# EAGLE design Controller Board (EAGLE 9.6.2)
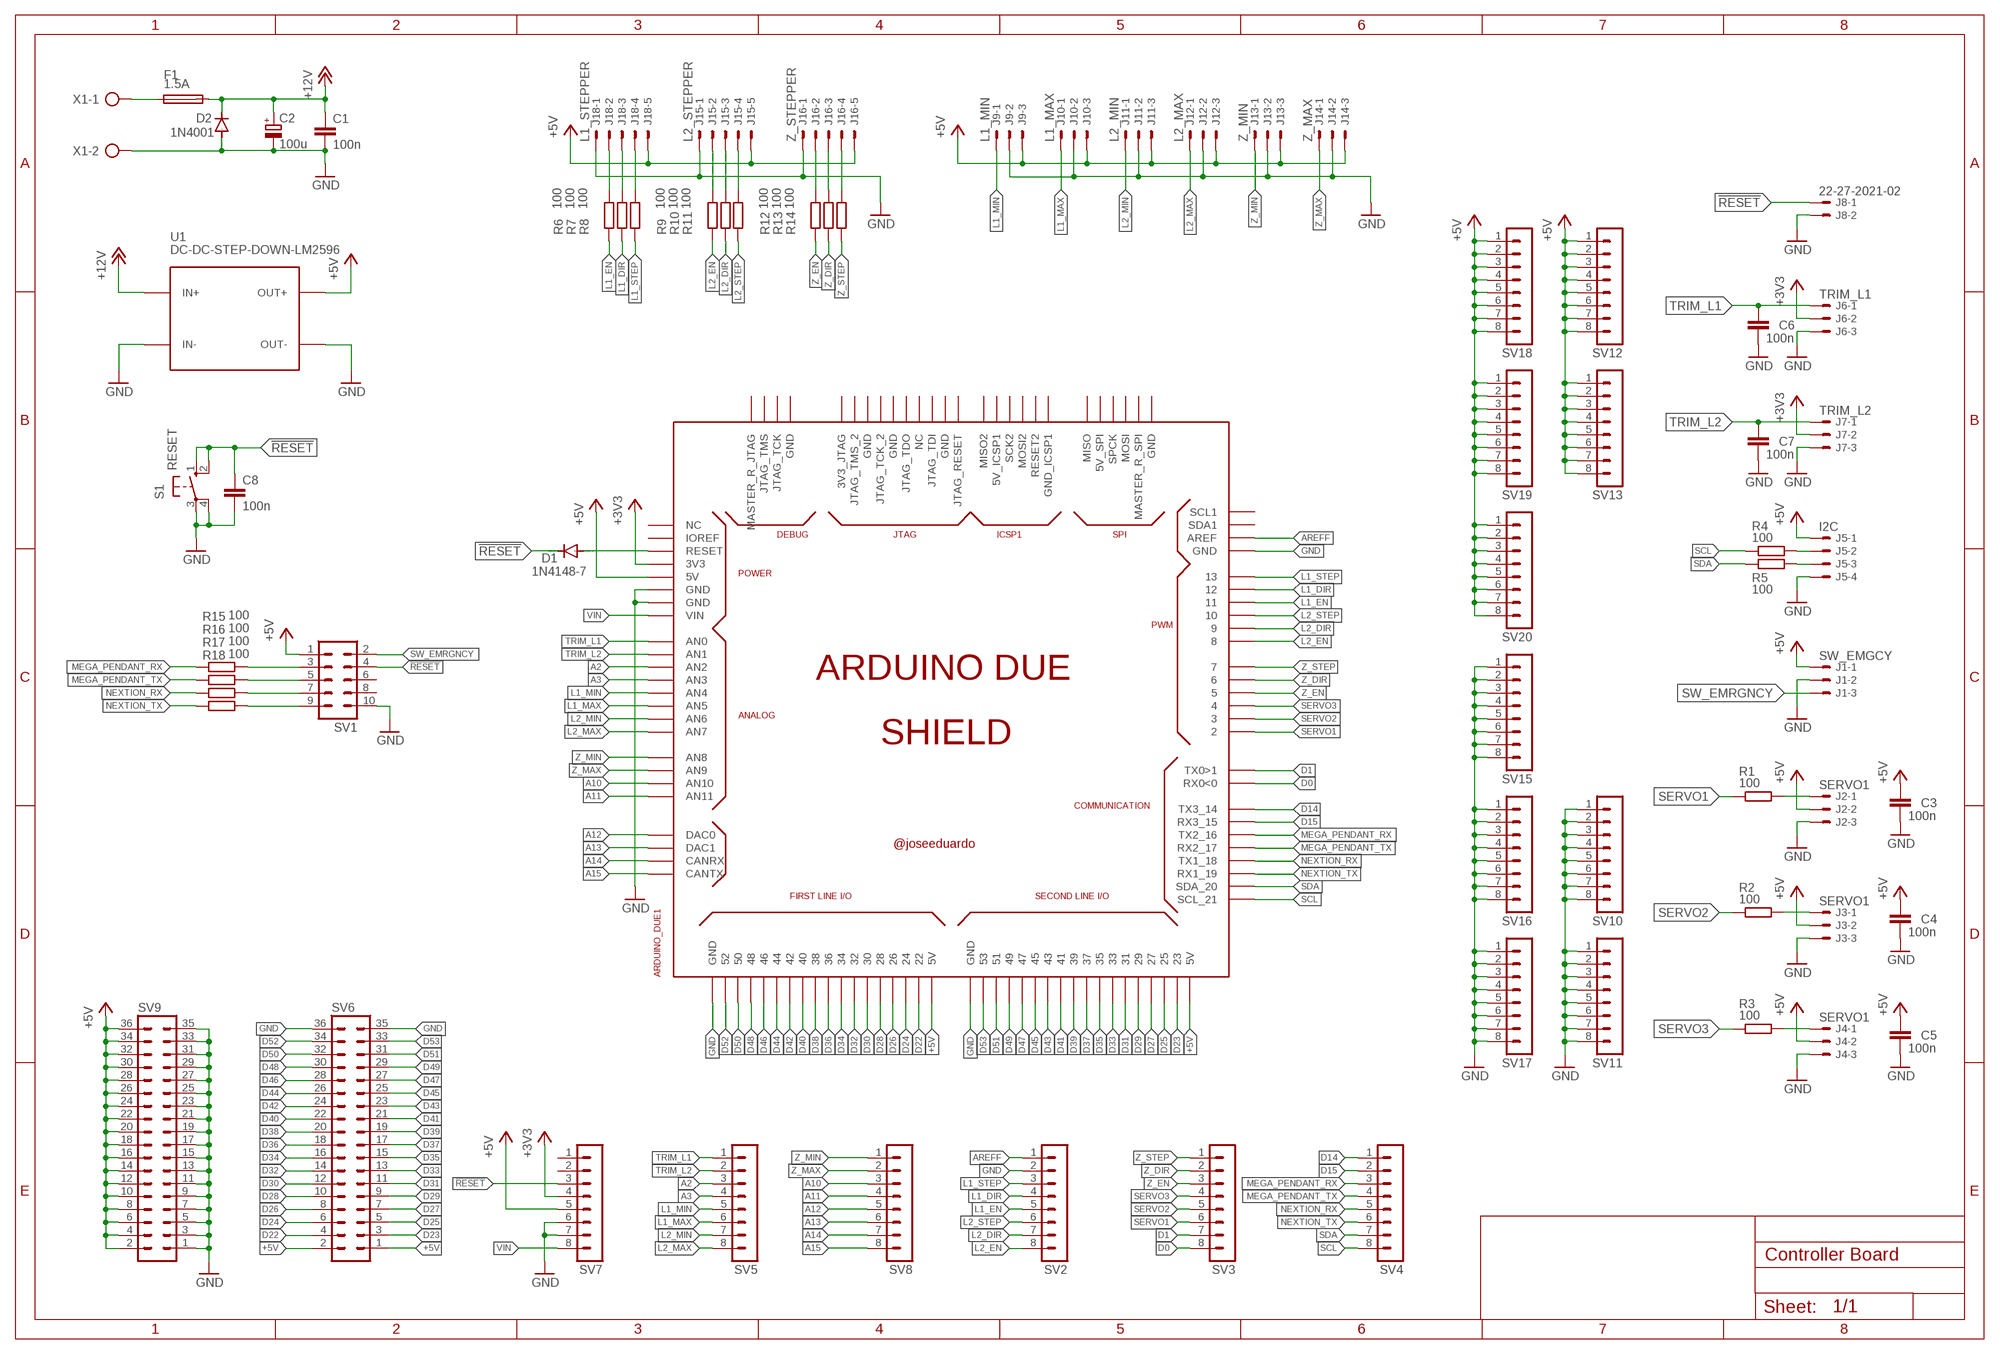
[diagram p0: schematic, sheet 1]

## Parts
ARDUINO_DUE1  ARDUINO_DUE_SHIELD_BTM  [ARDUINO_DUE_SHIELD_BOTTOM]
C1  100n  C-EU050-030X075  [C050-030X075]
C2  100u  CPOL-EUE3.5-8  [E3,5-8]
C3  100n  C-EU050-030X075  [C050-030X075]
C4  100n  C-EU050-030X075  [C050-030X075]
C5  100n  C-EU050-030X075  [C050-030X075]
C6  100n  C-EU050-030X075  [C050-030X075]
C7  100n  C-EU050-030X075  [C050-030X075]
C8  100n  C-EU050-030X075  [C050-030X075]
D1  1N4148-7  [DO35-7]
D2  1N4001  DIODE-DO41-7.6  [DO41-7.6]
F1  1.5A  SH22,5A  [SH22,5A]
J1  SW_EMGCY  22-27-2031-03  [6410-03]
J2  SERVO1  22-27-2031-03  [6410-03]
J3  SERVO1  22-27-2031-03  [6410-03]
J4  SERVO1  22-27-2031-03  [6410-03]
J5  I2C  22-27-2041-04  [6410-04]
J6  TRIM_L1  22-27-2031-03  [6410-03]
J7  TRIM_L2  22-27-2031-03  [6410-03]
J8  22-27-2021-02  [6410-02]
J9  L1_MIN  22-27-2031-03  [6410-03]
J10  L1_MAX  22-27-2031-03  [6410-03]
J11  L2_MIN  22-27-2031-03  [6410-03]
J12  L2_MAX  22-27-2031-03  [6410-03]
J13  Z_MIN  22-27-2031-03  [6410-03]
J14  Z_MAX  22-27-2031-03  [6410-03]
J15  L2_STEPPER  22-27-2051-05  [6410-05]
J16  Z_STEPPER  22-27-2051-05  [6410-05]
J18  L1_STEPPER  22-27-2051-05  [6410-05]
R1  100  R-EU_0207/7  [0207/7]
R2  100  R-EU_0207/7  [0207/7]
R3  100  R-EU_0207/7  [0207/7]
R4  100  R-EU_0207/7  [0207/7]
R5  100  R-EU_0207/7  [0207/7]
R6  100  R-EU_0207/7  [0207/7]
R7  100  R-EU_0207/7  [0207/7]
R8  100  R-EU_0207/7  [0207/7]
R9  100  R-EU_0207/7  [0207/7]
R10  100  R-EU_0207/7  [0207/7]
R11  100  R-EU_0207/7  [0207/7]
R12  100  R-EU_0207/7  [0207/7]
R13  100  R-EU_0207/7  [0207/7]
R14  100  R-EU_0207/7  [0207/7]
R15  100  R-EU_0207/7  [0207/7]
R16  100  R-EU_0207/7  [0207/7]
R17  100  R-EU_0207/7  [0207/7]
R18  100  R-EU_0207/7  [0207/7]
S1  RESET  10-XX  [B3F-10XX]
SV1  ML10  [ML10]
SV2  MA08-1  [MA08-1]
SV3  MA08-1  [MA08-1]
SV4  MA08-1  [MA08-1]
SV5  MA08-1  [MA08-1]
SV6  MA18-2  [MA18-2]
SV7  MA08-1  [MA08-1]
SV8  MA08-1  [MA08-1]
SV9  MA18-2  [MA18-2]
SV10  MA08-1  [MA08-1]
SV11  MA08-1  [MA08-1]
SV12  MA08-1  [MA08-1]
SV13  MA08-1  [MA08-1]
SV15  MA08-1  [MA08-1]
SV16  MA08-1  [MA08-1]
SV17  MA08-1  [MA08-1]
SV18  MA08-1  [MA08-1]
SV19  MA08-1  [MA08-1]
SV20  MA08-1  [MA08-1]
U1  DC-DC-STEP-DOWN-LM2596  [DC-DC-STEP-DOWN-LM2596]
X1  AK500/2  [AK500/2]

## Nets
!RESET: C8.1 D1.C J8.1 S1.1(S) S1.2(S1) SV1.4 SV7.3
+3V3: ARDUINO_DUE1.3V3 J6.2 J7.2 SV7.4
+5V: ARDUINO_DUE1.5V0(5V) ARDUINO_DUE1.5V0_1(5V) ARDUINO_DUE1.5V0_2(5V) C3.1 C4.1 C5.1 J1.1 J2.2 J3.2 J4.2 J5.1 J9.3 J10.3 J11.3 J12.3 J13.3 J14.3 J15.5 J16.5 J18.5 SV1.1 SV6.1 SV6.2 SV7.5 SV9.2 SV9.4 SV9.6 SV9.8 SV9.10 SV9.12 SV9.14 SV9.16 SV9.18 SV9.20 SV9.22 SV9.24 SV9.26 SV9.28 SV9.30 SV9.32 SV9.34 SV9.36 SV12.1 SV12.2 SV12.3 SV12.4 SV12.5 SV12.6 SV12.7 SV12.8 SV13.1 SV13.2 SV13.3 SV13.4 SV13.5 SV13.6 SV13.7 SV13.8 SV18.1 SV18.2 SV18.3 SV18.4 SV18.5 SV18.6 SV18.7 SV18.8 SV19.1 SV19.2 SV19.3 SV19.4 SV19.5 SV19.6 SV19.7 SV19.8 SV20.1 SV20.2 SV20.3 SV20.4 SV20.5 SV20.6 SV20.7 SV20.8 U1.OUT+
+12V: C1.1 C2.+ D2.C F1.2 U1.IN+
A2: ARDUINO_DUE1.A2(AN2) SV5.3
A3: ARDUINO_DUE1.A3(AN3) SV5.4
A10: ARDUINO_DUE1.A10(AN10) SV8.3
A11: ARDUINO_DUE1.A11(AN11) SV8.4
A12: ARDUINO_DUE1.DAC0 SV8.5
A13: ARDUINO_DUE1.DAC1 SV8.6
A14: ARDUINO_DUE1.CANRX SV8.7
A15: ARDUINO_DUE1.CANTX SV8.8
AREFF: ARDUINO_DUE1.AREF SV2.1
D0: ARDUINO_DUE1.0(RX0<0) SV3.8
D1: ARDUINO_DUE1.1(TX0>1) SV3.7
D14: ARDUINO_DUE1.14(TX3_14) SV4.1
D15: ARDUINO_DUE1.15(RX3_15) SV4.2
D22: ARDUINO_DUE1.22 SV6.4
D23: ARDUINO_DUE1.23 SV6.3
D24: ARDUINO_DUE1.24 SV6.6
D25: ARDUINO_DUE1.25 SV6.5
D26: ARDUINO_DUE1.26 SV6.8
D27: ARDUINO_DUE1.27 SV6.7
D28: ARDUINO_DUE1.28 SV6.10
D29: ARDUINO_DUE1.29 SV6.9
D30: ARDUINO_DUE1.30 SV6.12
D31: ARDUINO_DUE1.31 SV6.11
D32: ARDUINO_DUE1.32 SV6.14
D33: ARDUINO_DUE1.33 SV6.13
D34: ARDUINO_DUE1.34 SV6.16
D35: ARDUINO_DUE1.35 SV6.15
D36: ARDUINO_DUE1.36 SV6.18
D37: ARDUINO_DUE1.37 SV6.17
D38: ARDUINO_DUE1.38 SV6.20
D39: ARDUINO_DUE1.39 SV6.19
D40: ARDUINO_DUE1.40 SV6.22
D41: ARDUINO_DUE1.41 SV6.21
D42: ARDUINO_DUE1.42 SV6.24
D43: ARDUINO_DUE1.43 SV6.23
D44: ARDUINO_DUE1.44 SV6.26
D45: ARDUINO_DUE1.45 SV6.25
D46: ARDUINO_DUE1.46 SV6.28
D47: ARDUINO_DUE1.47 SV6.27
D48: ARDUINO_DUE1.48 SV6.30
D49: ARDUINO_DUE1.49 SV6.29
D50: ARDUINO_DUE1.50 SV6.32
D51: ARDUINO_DUE1.51 SV6.31
D52: ARDUINO_DUE1.52 SV6.34
D53: ARDUINO_DUE1.53 SV6.33
GND: ARDUINO_DUE1.GND ARDUINO_DUE1.GND_1(GND) ARDUINO_DUE1.GND_2(GND) ARDUINO_DUE1.GND_3(GND) ARDUINO_DUE1.GND_4(GND) C1.2 C2.- C3.2 C4.2 C5.2 C6.2 C7.2 C8.2 D2.A J1.2 J2.3 J3.3 J4.3 J5.4 J6.3 J7.3 J8.2 J9.2 J10.2 J11.2 J12.2 J13.2 J14.2 J15.1 J16.1 J18.1 S1.3(P) S1.4(P1) SV1.10 SV2.2 SV6.35 SV6.36 SV7.6 SV7.7 SV9.1 SV9.3 SV9.5 SV9.7 SV9.9 SV9.11 SV9.13 SV9.15 SV9.17 SV9.19 SV9.21 SV9.23 SV9.25 SV9.27 SV9.29 SV9.31 SV9.33 SV9.35 SV10.1 SV10.2 SV10.3 SV10.4 SV10.5 SV10.6 SV10.7 SV10.8 SV11.1 SV11.2 SV11.3 SV11.4 SV11.5 SV11.6 SV11.7 SV11.8 SV15.1 SV15.2 SV15.3 SV15.4 SV15.5 SV15.6 SV15.7 SV15.8 SV16.1 SV16.2 SV16.3 SV16.4 SV16.5 SV16.6 SV16.7 SV16.8 SV17.1 SV17.2 SV17.3 SV17.4 SV17.5 SV17.6 SV17.7 SV17.8 U1.IN- U1.OUT- X1.2
L1_DIR: ARDUINO_DUE1.12 R7.1 SV2.4
L1_EN: ARDUINO_DUE1.11 R6.1 SV2.5
L1_MAX: ARDUINO_DUE1.A5(AN5) J10.1 SV5.6
L1_MIN: ARDUINO_DUE1.A4(AN4) J9.1 SV5.5
L1_STEP: ARDUINO_DUE1.13 R8.1 SV2.3
L2_DIR: ARDUINO_DUE1.9 R10.1 SV2.7
L2_EN: ARDUINO_DUE1.8 R9.1 SV2.8
L2_MAX: ARDUINO_DUE1.A7(AN7) J12.1 SV5.8
L2_MIN: ARDUINO_DUE1.A6(AN6) J11.1 SV5.7
L2_STEP: ARDUINO_DUE1.10 R11.1 SV2.6
MEGA_PENDANT_RX: ARDUINO_DUE1.16(TX2_16) R15.1 SV4.3
MEGA_PENDANT_TX: ARDUINO_DUE1.17(RX2_17) R16.1 SV4.4
N$1: ARDUINO_DUE1.RESET D1.A
N$2: F1.1 X1.1
N$3: J2.1 R1.2
N$4: J3.1 R2.2
N$5: J4.1 R3.2
N$6: J5.2 R4.2
N$7: J5.3 R5.2
N$8: J18.2 R6.2
N$9: J18.3 R7.2
N$10: J18.4 R8.2
N$11: J15.2 R9.2
N$12: J15.3 R10.2
N$13: J15.4 R11.2
N$14: J16.4 R14.2
N$15: J16.3 R13.2
N$16: J16.2 R12.2
N$17: R15.2 SV1.3
N$18: R16.2 SV1.5
N$19: R17.2 SV1.7
N$20: R18.2 SV1.9
NEXTION_RX: ARDUINO_DUE1.18(TX1_18) R17.1 SV4.5
NEXTION_TX: ARDUINO_DUE1.19(RX1_19) R18.1 SV4.6
SCL: ARDUINO_DUE1.21(SCL_21) R4.1 SV4.8
SDA: ARDUINO_DUE1.20(SDA_20) R5.1 SV4.7
SERVO1: ARDUINO_DUE1.2 R1.1 SV3.6
SERVO2: ARDUINO_DUE1.3 R2.1 SV3.5
SERVO3: ARDUINO_DUE1.4 R3.1 SV3.4
SW_EMRGNCY: J1.3 SV1.2
TRIM_L1: ARDUINO_DUE1.A0(AN0) C6.1 J6.1 SV5.1
TRIM_L2: ARDUINO_DUE1.A1(AN1) C7.1 J7.1 SV5.2
VIN: ARDUINO_DUE1.VIN SV7.8
Z_DIR: ARDUINO_DUE1.6 R13.1 SV3.2
Z_EN: ARDUINO_DUE1.5 R12.1 SV3.3
Z_MAX: ARDUINO_DUE1.A9(AN9) J14.1 SV8.2
Z_MIN: ARDUINO_DUE1.A8(AN8) J13.1 SV8.1
Z_STEP: ARDUINO_DUE1.7 R14.1 SV3.1
Unconnected: ARDUINO_DUE1.3V3_JTAG ARDUINO_DUE1.5V_2(5V_SPI) ARDUINO_DUE1.5V_ICSP1 ARDUINO_DUE1.GND_5(GND) ARDUINO_DUE1.GND_7(GND) ARDUINO_DUE1.GND_8(GND) ARDUINO_DUE1.GND_9(GND) ARDUINO_DUE1.GND_10(GND) ARDUINO_DUE1.GND_ICSP1 ARDUINO_DUE1.IOREF ARDUINO_DUE1.JTAG_RESET ARDUINO_DUE1.JTAG_TCK ARDUINO_DUE1.JTAG_TCK_2 ARDUINO_DUE1.JTAG_TDI ARDUINO_DUE1.JTAG_TDO ARDUINO_DUE1.JTAG_TMS ARDUINO_DUE1.JTAG_TMS_2 ARDUINO_DUE1.MASTER_RESET_JTAG(MASTER_R_JTAG) ARDUINO_DUE1.MASTER_RESET_SPI(MASTER_R_SPI) ARDUINO_DUE1.MISO ARDUINO_DUE1.MISO2 ARDUINO_DUE1.MOSI ARDUINO_DUE1.MOSI2 ARDUINO_DUE1.NC_2(NC) ARDUINO_DUE1.NC_5(NC) ARDUINO_DUE1.RESET2 ARDUINO_DUE1.SCK2 ARDUINO_DUE1.SCL1 ARDUINO_DUE1.SDA1 ARDUINO_DUE1.SPCK SV1.6 SV1.8 SV7.1 SV7.2

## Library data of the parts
ARDUINO_DUE1 = arduino_due_shield:ARDUINO_DUE_SHIELD
C1 C3-C8 = rcl:C-EU: CAPACITOR, European symbol; SPICEPREFIX: C
C2 = rcl:CPOL-EU: POLARIZED CAPACITOR, European symbol; SPICEPREFIX: C
D1 = diode:1N4148: DIODE
D2 = diode:DIODE-: DIODE
F1 = Khoirul_Component:SH22,5A: FUSE HOLDER
J1-J4 J6 J7 J9-J14 = con-molex:22-?-03: CONNECTOR wire to board 2.54 mm (.1 inch) pitch header; MF: MOLEX; OC_FARNELL: unknown; OC_NEWARK: unknown
J5 = con-molex:22-?-04: CONNECTOR wire to board 2.54 mm (.1 inch) pitch header; MF: MOLEX; OC_FARNELL: unknown; OC_NEWARK: unknown
J8 = con-molex:22-?-02: CONNECTOR; MF: MOLEX; OC_FARNELL: unknown; OC_NEWARK: unknown
J15 J16 J18 = con-molex:22-?-05: CONNECTOR wire to board 2.54 mm (.1 inch) pitch header; MF: MOLEX; OC_FARNELL: unknown; OC_NEWARK: unknown
R1-R18 = rcl:R-EU_: RESISTOR, European symbol; SPICEPREFIX: R
S1 = switch-omron:10-XX: OMRON SWITCH; MPN: B3F-1000; OC_FARNELL: 176432; OC_NEWARK: 36M3542
SV1 = con-ml:ML10: HARTING; OC_FARNELL: unknown; OC_NEWARK: unknown
SV2-SV5 SV7 SV8 SV10-SV13 SV15-SV20 = con-lstb:MA08-1: PIN HEADER; OC_FARNELL: unknown; OC_NEWARK: unknown
SV6 SV9 = con-lstb:MA18-2: PIN HEADER; OC_FARNELL: unknown; OC_NEWARK: unknown
U1 = diy-modules:DC-DC-STEP-DOWN-LM2596: DC/DC Step-Down Regulator based on LM2596-ADJ chip LM2596 datasheet available here: http://www.ti.com/lit/ds/symlink/lm2596.pdf Click here to find device on ebay.com
X1 = con-ptr500:AK500/2: CONNECTOR; OC_FARNELL: unknown; OC_NEWARK: unknown

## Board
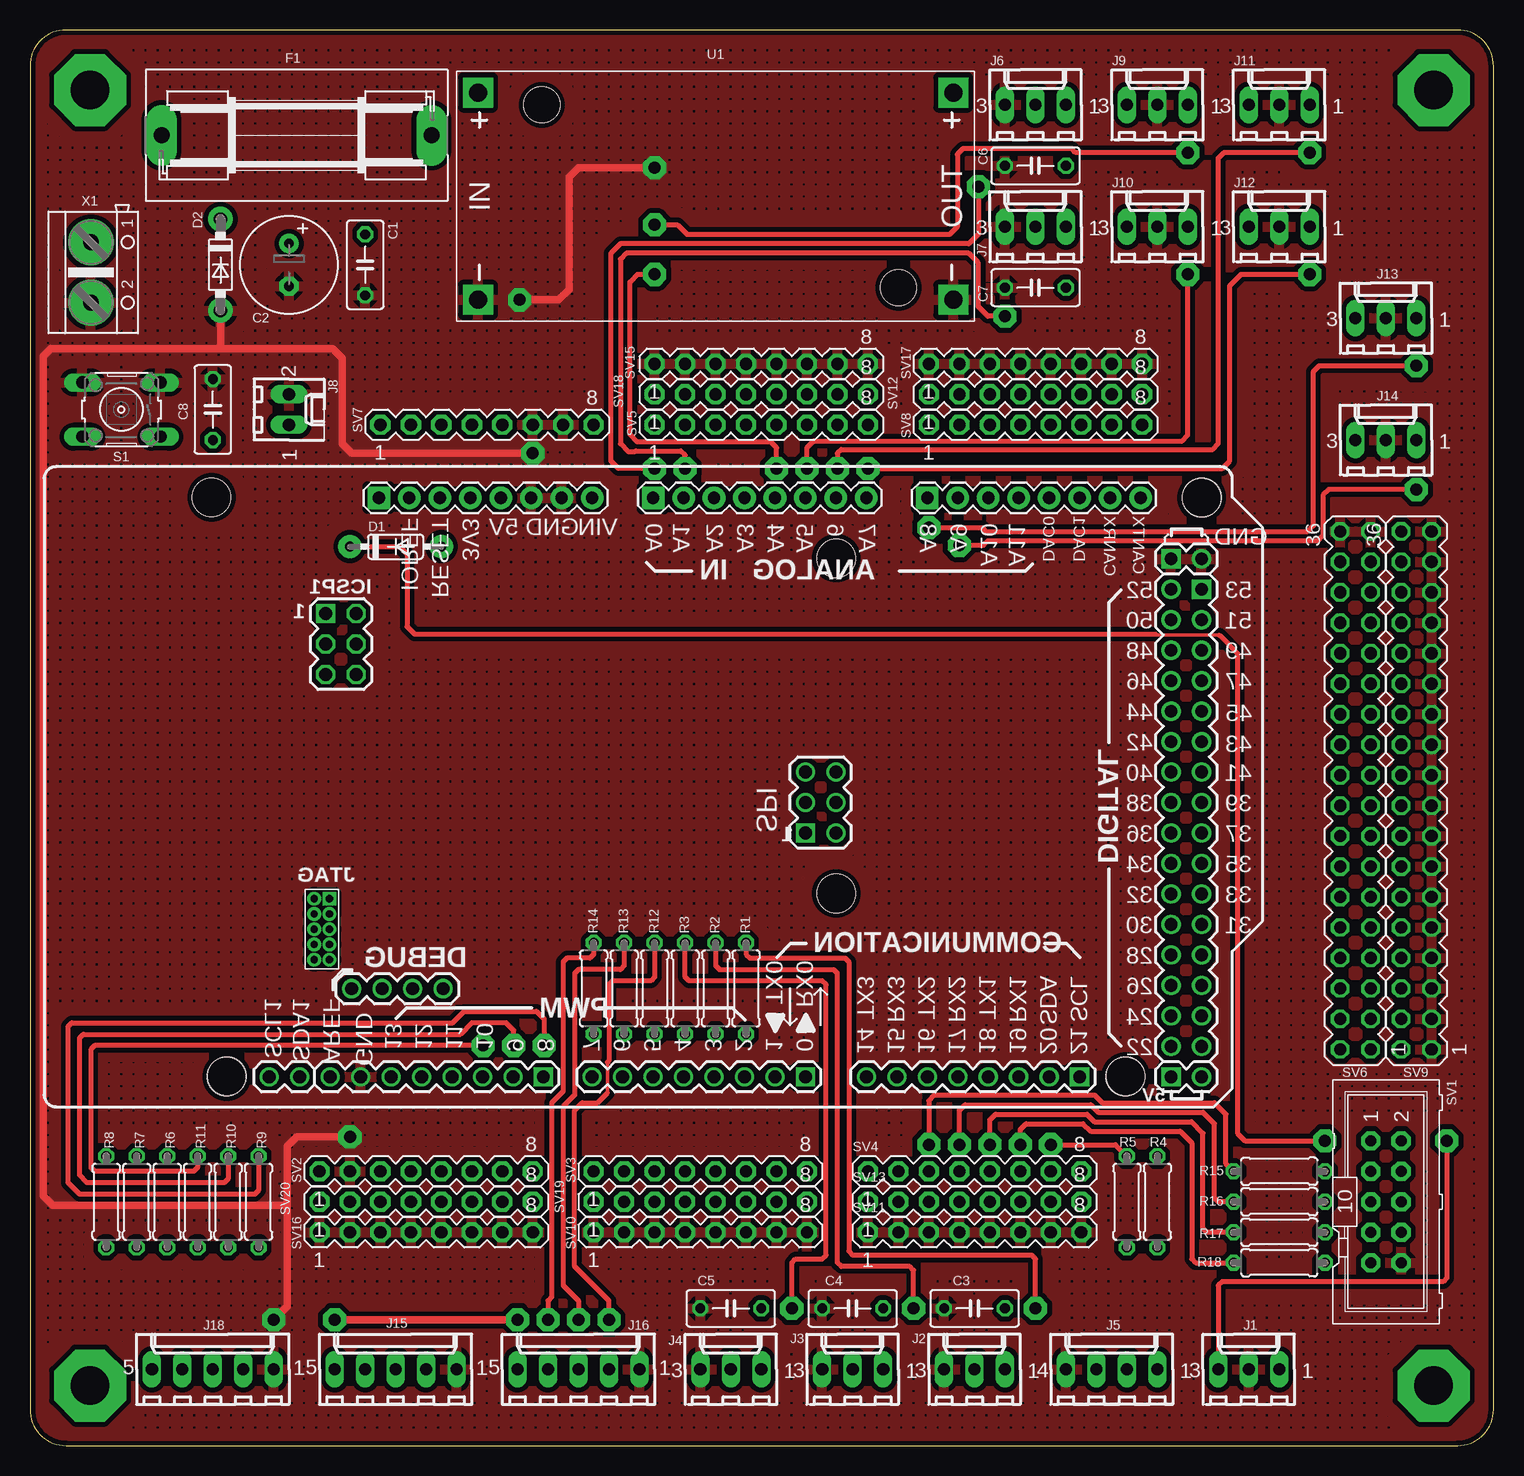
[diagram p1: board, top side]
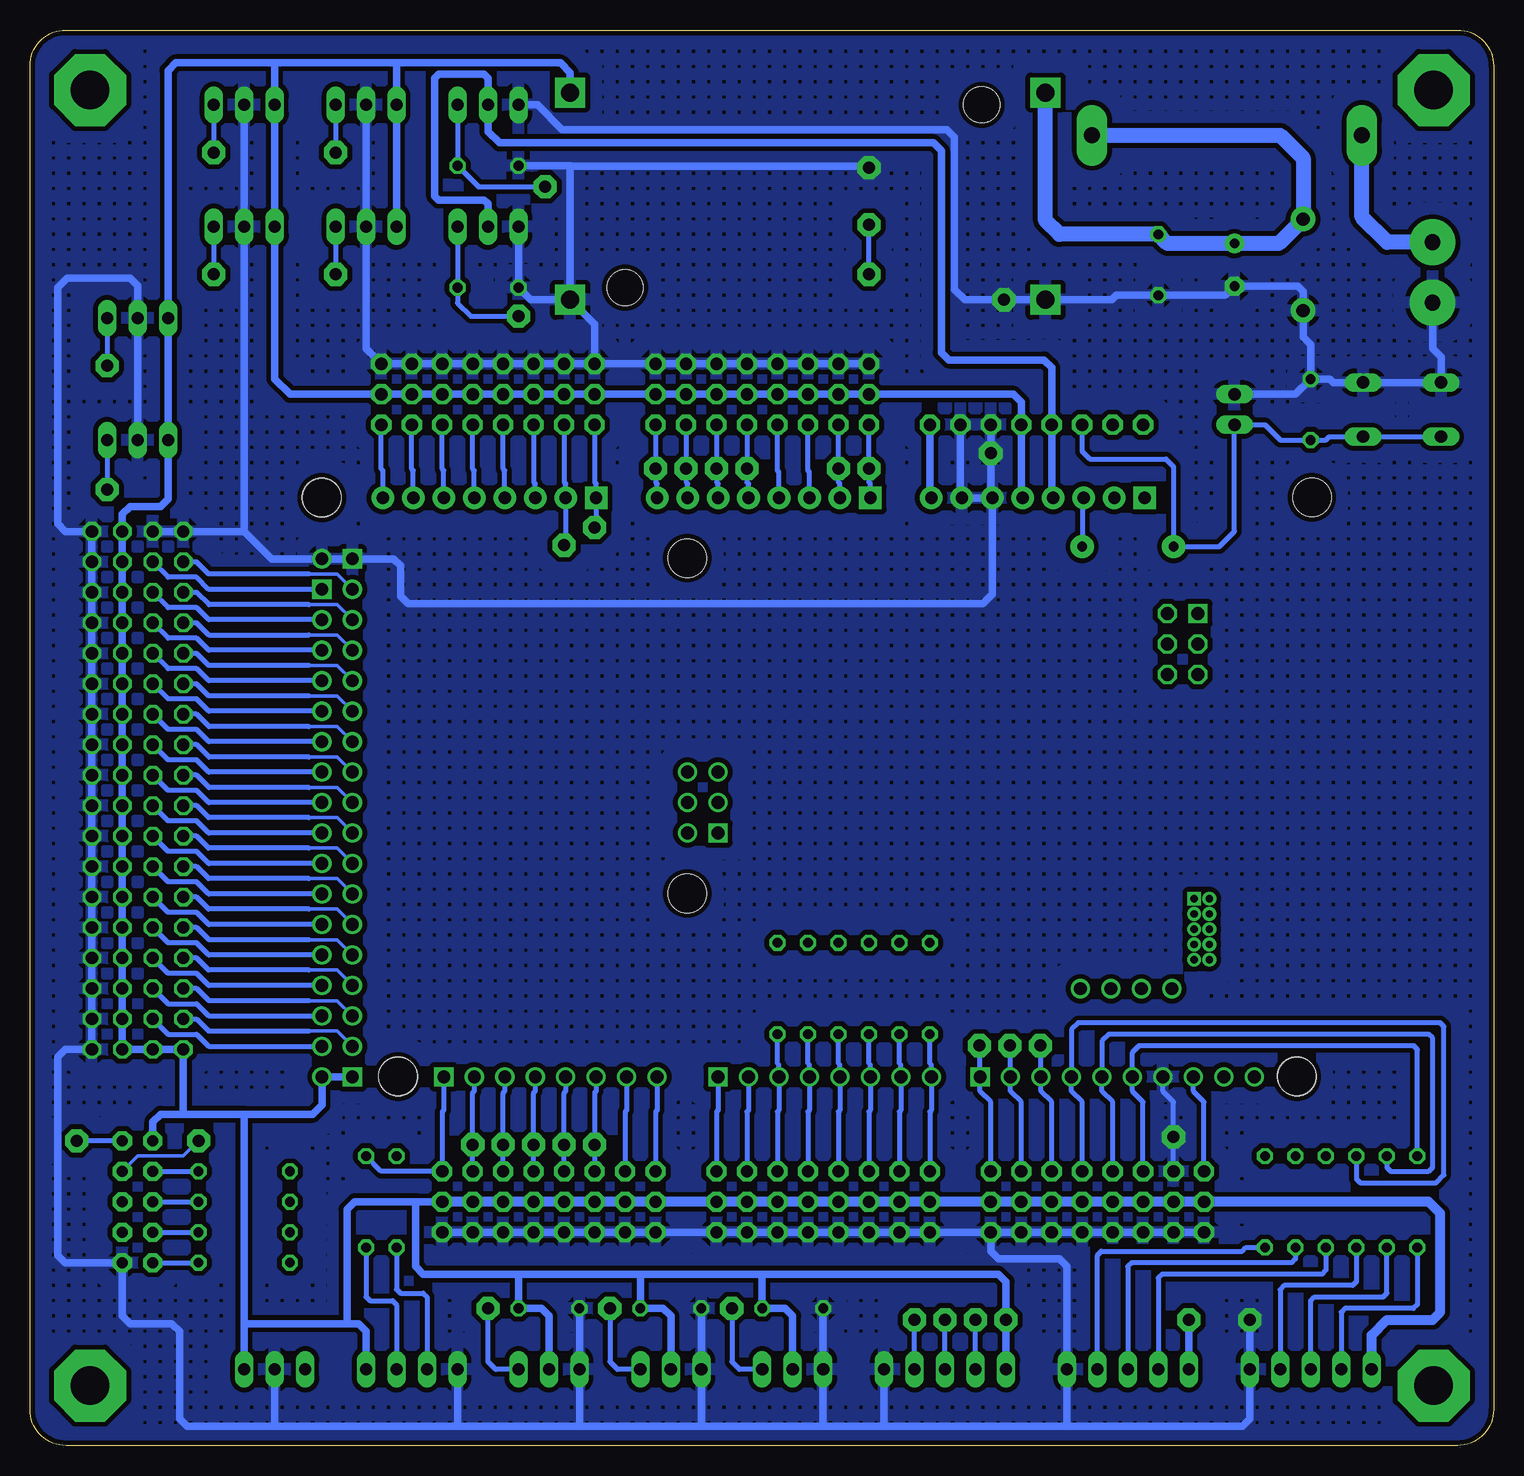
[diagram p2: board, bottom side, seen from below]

Size 122 x 118 mm. Coordinates in mm from the lower left corner, seen from the top.
Outline: 122,3 122,115 arc90 119,118 3,118 arc90 0,115 0,3 arc90 3,0 119,0 arc90 122,3
Copper layers (1*16): Top 0.035mm / dielectric 1.5mm / Bottom 0.035mm
Design rules "default": minimum track width 12mil, minimum drill 0.8mm, track to track 12mil, track to pad 12mil, pad to pad 12mil, via to via 12mil, smd to smd 12mil, copper to edge 12mil, drill to drill 6mil, minimum pad ring 10mil, minimum via ring 8mil, stop-mask expansion 12mil, vias tented up to drill 0mil, thermal gap 16mil

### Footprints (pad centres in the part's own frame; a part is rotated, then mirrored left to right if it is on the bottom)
ARDUINO_DUE_SHIELD_BOTTOM = drill 1.067 square: 0 63.373,51.816; 5V0_1 93.853,51.816; 8 41.529,51.816; 21 86.233,51.816; 53 96.393,11.176; GND_2 93.853,8.636; MISO 63.373,31.496; MISO2 23.384,13.196 | drill 1.067: 1 60.833,51.816; 2 58.293,51.816; 3 55.753,51.816; 4 53.213,51.816; 5 50.673,51.816; 5V0_2 96.393,51.816; 5V_2 65.913,31.496; 6 48.133,51.816; 7 45.593,51.816; 9 38.989,51.816; 10 36.449,51.816; 11 33.909,51.816; 12 31.369,51.816; 13 28.829,51.816; 14 68.453,51.816; 15 70.993,51.816; 16 73.533,51.816; 17 76.073,51.816; 18 78.613,51.816; 19 81.153,51.816; 20 83.693,51.816; 22 93.853,49.276; 23 96.393,49.276; 24 93.853,46.736; 25 96.393,46.736; 26 93.853,44.196; 27 96.393,44.196; 28 93.853,41.656; 29 96.393,41.656; 30 93.853,39.116; 31 96.393,39.116; 32 93.853,36.576; 33 96.393,36.576; 34 93.853,34.036; 35 96.393,34.036; 36 93.853,31.496; 37 96.393,31.496; 38 93.853,28.956; 39 96.393,28.956; 40 93.853,26.416; 41 96.393,26.416; 42 93.853,23.876; 43 96.393,23.876; 44 93.853,21.336; 45 96.393,21.336; 46 93.853,18.796; 47 96.393,18.796; 48 93.853,16.256; 49 96.393,16.256; 50 93.853,13.716; 51 96.393,13.716; 52 93.853,11.176; AREF 23.749,51.816; GND_3 96.393,8.636; GND_4 26.289,51.816; GND_5 65.913,26.416; GND_7 33.161,44.473; JTAG_TCK 30.621,44.473; JTAG_TMS 28.081,44.473; MASTER_RESET_JTAG 25.541,44.473; MASTER_RESET_SPI 63.373,26.416; MOSI 65.913,28.956; SCL1 18.669,51.816; SDA1 21.209,51.816; SPCK 63.373,28.956 | drill 1.016 pad 1.88: 3V3 35.433,3.556; 5V0 37.973,3.556; A1 53.213,3.556; A2 55.753,3.556; A3 58.293,3.556; A4 60.833,3.556; A5 63.373,3.556; A6 65.913,3.556; A7 68.453,3.556; A9 76.073,3.556; A10 78.613,3.556; A11 81.153,3.556; CANRX 88.773,3.556; CANTX 91.313,3.556; DAC0 83.693,3.556; DAC1 86.233,3.556; GND 40.513,3.556; GND_1 43.053,3.556; IOREF 30.346,3.543; RESET 32.893,3.555; VIN 45.593,3.556 | drill 0.6 pad 1.016 square: 3V3_JTAG 23.689,36.964 | drill 1.067 octagon: 5V_ICSP1 25.924,13.196; GND_ICSP1 25.924,18.276; MOSI2 25.924,15.736; RESET2 23.384,18.276; SCK2 23.384,15.736 | drill 1.016 pad 1.88 square: A0 50.673,3.556; A8 73.533,3.556; NC_2 27.806,3.543 | drill 0.6 pad 1.143: GND_8 23.689,38.234; GND_9 23.689,40.774; GND_10 23.689,42.044; JTAG_RESET 22.419,42.044; JTAG_TCK_2 22.419,38.234; JTAG_TDI 22.419,40.774; JTAG_TDO 22.419,39.504; JTAG_TMS_2 22.419,36.964; NC_5 23.689,39.504 | hole 3.2: 15.113,51.816; 90.043,51.816; 96.393,3.556; 96.418,3.505; 15.138,51.765; 90.068,51.765; 13.868,3.505; 65.938,36.525; 65.938,8.585
C050-030X075 = drill 0.813 octagon: 1 -2.54,0; 2 2.54,0
E3,5-8 = drill 0.813 pad 1.6: + -1.778,0 | drill 0.813 pad 1.6 octagon: - 1.778,0
DO35-7 = drill 0.813 pad 1.93: A 3.81,0; C -3.81,0
DO41-7.6 = drill 1.1 pad 2.032: A 3.81,0; C -3.81,0
SH22,5A = drill 1.321 pad 2.54 long: 1 -11.252,0; 2 11.252,0
6410-03 = drill 1.016 long: 1 2.54,0; 2 0,0; 3 -2.54,0
6410-04 = drill 1.016 long: 1 3.81,0; 2 1.27,0; 3 -1.27,0; 4 -3.81,0
6410-02 = drill 1.016 long: 1 1.27,0; 2 -1.27,0
6410-05 = drill 1.016 long: 1 5.08,0; 2 2.54,0; 3 0,0; 4 -2.54,0; 5 -5.08,0
0207/7 = drill 0.813 octagon: 1 -3.81,0; 2 3.81,0
B3F-10XX = drill 1.016 long: 1 -3.251,2.261; 2 3.251,2.261; 3 -3.251,-2.261; 4 3.251,-2.261
ML10 = drill 0.914 pad 1.6 octagon: 1 -5.08,-1.27; 2 -5.08,1.27; 3 -2.54,-1.27; 4 -2.54,1.27; 5 0,-1.27; 6 0,1.27; 7 2.54,-1.27; 8 2.54,1.27; 9 5.08,-1.27; 10 5.08,1.27
MA08-1 = drill 1.016 pad 1.676 octagon: 1 -8.89,0; 2 -6.35,0; 3 -3.81,0; 4 -1.27,0; 5 1.27,0; 6 3.81,0; 7 6.35,0; 8 8.89,0
MA18-2 = drill 1.016 octagon: 1 -21.59,-1.27; 2 -21.59,1.27; 3 -19.05,-1.27; 4 -19.05,1.27; 5 -16.51,-1.27; 6 -16.51,1.27; 7 -13.97,-1.27; 8 -13.97,1.27; 9 -11.43,-1.27; 10 -11.43,1.27; 11 -8.89,-1.27; 12 -8.89,1.27; 13 -6.35,-1.27; 14 -6.35,1.27; 15 -3.81,-1.27; 16 -3.81,1.27; 17 -1.27,-1.27; 18 -1.27,1.27; 19 1.27,-1.27; 20 1.27,1.27; 21 3.81,-1.27; 22 3.81,1.27; 23 6.35,-1.27; 24 6.35,1.27; 25 8.89,-1.27; 26 8.89,1.27; 27 11.43,-1.27; 28 11.43,1.27; 29 13.97,-1.27; 30 13.97,1.27; 31 16.51,-1.27; 32 16.51,1.27; 33 19.05,-1.27; 34 19.05,1.27; 35 21.59,-1.27; 36 21.59,1.27
DC-DC-STEP-DOWN-LM2596 = drill 1.5 pad 2.5 square: IN+ -19.812,8.636; IN- -19.812,-8.636; OUT+ 19.812,8.636; OUT- 19.812,-8.636 | hole 3: -14.478,7.62; 15.24,-7.62
AK500/2 = drill 1.321 pad 3.81: 1 -2.515,0; 2 2.515,0

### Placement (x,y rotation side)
ARDUINO_DUE1  1.27,82.55 180 bottom
C1  27.94,98.42 270 top
C2  21.59,98.42 270 top
C3  78.74,11.43 180 top
C4  68.58,11.43 180 top
C5  58.42,11.43 180 top
C6  83.82,106.68 180 top
C7  83.82,96.52 180 top
C8  15.24,86.36 90 top
D1  30.48,74.93 0 top
D2  15.88,98.42 270 top
F1  22.23,109.22 0 top
J1  101.6,6.35 0 top
J2  78.74,6.35 0 top
J3  68.58,6.35 0 top
J4  58.42,6.35 0 top
J5  90.17,6.35 0 top
J6  83.82,111.76 0 top
J7  83.82,101.6 0 top
J8  21.59,86.36 270 top
J9  93.98,111.76 0 top
J10  93.98,101.6 0 top
J11  104.14,111.76 0 top
J12  104.14,101.6 0 top
J13  113.03,93.98 0 top
J14  113.03,83.82 0 top
J15  30.48,6.35 0 top
J16  45.72,6.35 0 top
J18  15.24,6.35 0 top
R1  59.69,38.1 90 top
R2  57.15,38.1 90 top
R3  54.61,38.1 90 top
R4  93.98,20.32 270 top
R5  91.44,20.32 270 top
R6  11.43,20.32 270 top
R7  8.89,20.32 270 top
R8  6.35,20.32 270 top
R9  19.05,20.32 270 top
R10  16.51,20.32 270 top
R11  13.97,20.32 270 top
R12  52.07,38.1 90 top
R13  49.53,38.1 90 top
R14  46.99,38.1 90 top
R15  104.14,22.86 0 top
R16  104.14,20.32 0 top
R17  104.14,17.78 0 top
R18  104.14,15.24 0 top
S1  7.62,86.36 180 top
SV1  113.03,20.32 270 top
SV2  33.02,22.86 0 top
SV3  55.88,22.86 0 top
SV4  78.74,22.86 0 top
SV5  60.96,85.09 0 top
SV6  110.49,54.61 90 top
SV7  38.1,85.09 0 top
SV8  83.82,85.09 0 top
SV9  115.57,54.61 90 top
SV10  55.88,17.78 0 top
SV11  78.74,17.78 0 top
SV12  83.82,87.63 0 top
SV13  78.74,20.32 0 top
SV15  60.96,90.17 0 top
SV16  33.02,17.78 0 top
SV17  83.82,90.17 0 top
SV18  60.96,87.63 0 top
SV19  55.88,20.32 0 top
SV20  33.02,20.32 0 top
U1  57.15,104.14 0 top
X1  5.08,97.79 270 top

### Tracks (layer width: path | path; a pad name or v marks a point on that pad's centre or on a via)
!RESET  (via drill 1 pad 1.93)
  Top 0.305: 93.82,67.63 93.9,67.55 99.14,67.55
  Top 0.406: 93.82,67.63 32.07,67.63 31.43,68.26 31.43,74.3 30.8,74.93 D1.C | 99.14,67.55 100.65,66.04 100.65,26.04 101.28,25.4 v107.95,25.4
  Bottom 0.305: SV1.4 113.03,24.13 109.22,24.13 v107.95,25.4
  Bottom 0.406: S1.2 S1.1 13.69,84.1 13.97,83.82 C8.1 17.78,83.82 19.05,85.09 J8.1 21.59,76.2 22.86,74.93 D1.C 26.67,81.6 27.3,82.23 33.66,82.23 34.29,82.87 SV7.3
+3V3
  Bottom 0.61: ARDUINO_DUE1.3V3 36.83,79.12 SV7.4 36.83,89.85 37.47,90.49 45.4,90.49 46.04,91.12 46.04,107.95 46.67,108.58 82.87,108.58 83.82,109.54 J6.2 83.82,113.98 84.14,114.3 87.95,114.3 88.27,113.98 88.27,104.14 87.95,103.82 84.14,103.82 83.82,103.5 J7.2
+5V  (via drill 1 pad 1.93)
  Top 0.61: v25.4,10.48 v40.64,10.48
  Bottom 0.61: ARDUINO_DUE1.5V0 39.37,79.12 SV7.5 39.37,87 40.01,87.63 SV18.1 SV18.2 SV18.3 SV18.4 SV18.5 SV18.6 SV18.7 SV18.8 SV12.1 SV12.2 SV12.3 SV12.4 SV12.5 SV12.6 SV12.7 SV12.8 100.33,87.63 101.6,88.9 J12.3 J11.3 101.6,115.25 | U1.OUT+ 76.96,114.43 77.79,115.25 91.44,115.25 | 91.44,115.25 101.6,115.25 | 101.6,115.25 109.86,115.25 110.49,114.62 J13.3 J14.3 110.49,78.9 111.12,78.26 113.67,78.26 114.3,77.63 SV9.36 SV9.34 SV9.32 SV9.30 SV9.28 SV9.26 SV9.24 SV9.22 SV9.20 SV9.18 SV9.16 SV9.14 SV9.12 SV9.10 SV9.8 SV9.6 SV9.4 SV9.2 SV6.1 SV6.2 109.22,27.62 | ARDUINO_DUE1.5V0_1 ARDUINO_DUE1.5V0_2 97.66,28.38 98.42,27.62 104.14,27.62 | SV1.1 111.76,26.99 111.12,27.62 109.22,27.62 | J4.2 58.42,10.79 59.05,11.43 C5.1 60.96,14.29 | J3.2 68.58,10.79 69.22,11.43 C4.1 71.12,14.29 | J2.2 78.74,10.79 79.38,11.43 C3.1 81.28,14.29 | J15.5 v25.4,10.48 | J16.5 v40.64,10.48 40.64,13.65 41.27,14.29 60.96,14.29 | 60.96,14.29 71.12,14.29 | 71.12,14.29 81.28,14.29 | J5.1 93.98,9.53 94.61,10.16 95.57,10.16 | 95.57,10.16 104.14,10.16 | J1.1 104.14,10.16 | 81.28,14.29 89.22,14.29 89.85,14.92 89.85,20.32 | 95.57,10.16 95.57,19.68 94.93,20.32 89.85,20.32 | 89.85,20.32 SV13.8 | 104.14,10.16 104.14,27.62 | 104.14,27.62 109.22,27.62 | 91.44,115.25 J9.3 J10.3
  Bottom 0.813: J18.5 10.16,9.21 8.89,10.48 5.08,10.48 4.45,11.11 4.45,19.37 5.4,20.32 SV20.1 SV20.2 SV20.3 SV20.4 SV20.5 SV20.6 SV20.7 SV20.8 SV19.1 SV19.2 SV19.3 SV19.4 SV19.5 SV19.6 SV19.7 SV19.8 SV13.1 SV13.2 SV13.3 SV13.4 SV13.5 SV13.6 SV13.7 SV13.8
+12V
  Bottom 1.27: F1.2 17.78,109.22 15.88,107.31 D2.C 17.91,100.2 C2.+ 27.18,100.2 C1.1 36.2,100.97 37.34,102.11 U1.IN+
A2
  Bottom 0.406: ARDUINO_DUE1.A2 57.02,81.15 57.15,81.28 SV5.3
A3
  Bottom 0.406: ARDUINO_DUE1.A3 59.56,81.15 59.69,81.28 SV5.4
A10
  Bottom 0.406: ARDUINO_DUE1.A10 79.88,80.17 80.01,80.3 SV8.3
A11
  Bottom 0.406: ARDUINO_DUE1.A11 82.42,81.28 82.55,81.41 SV8.4
A12
  Bottom 0.406: ARDUINO_DUE1.DAC0 84.96,81.28 85.09,81.41 SV8.5
A13
  Bottom 0.406: ARDUINO_DUE1.DAC1 87.5,81.28 87.63,81.41 SV8.6
A14
  Bottom 0.406: ARDUINO_DUE1.CANRX 90.04,81.28 90.17,81.41 SV8.7
A15
  Bottom 0.406: ARDUINO_DUE1.CANTX 92.58,81.28 92.71,81.41 SV8.8
AREFF
  Bottom 0.406: ARDUINO_DUE1.AREF 25.02,29.53 24.13,28.64 SV2.1
D0
  Bottom 0.406: ARDUINO_DUE1.0 64.64,27.94 64.77,27.81 SV3.8
D1
  Bottom 0.406: ARDUINO_DUE1.1 62.1,27.94 62.23,27.81 SV3.7
D14
  Bottom 0.406: ARDUINO_DUE1.14 69.72,27.94 69.85,27.81 SV4.1
D15
  Bottom 0.406: ARDUINO_DUE1.15 72.26,27.94 72.39,27.81 SV4.2
D22
  Bottom 0.305: ARDUINO_DUE1.22 96.41,34.56 98.74,34.56 | 107.16,34.61 107.11,34.56
  Bottom 0.406: SV6.4 108.11,35.56 107.16,34.61 | 107.11,34.56 98.74,34.56
D23
  Bottom 0.406: SV6.3 110.49,34.29 108.11,34.29 107.09,33.27 ARDUINO_DUE1.23
D24
  Bottom 0.305: ARDUINO_DUE1.24 96.38,37.07 98.74,37.07
  Bottom 0.406: 98.74,37.07 107.08,37.07 108.11,38.1 SV6.6
D25
  Bottom 0.406: SV6.5 110.49,36.83 108.11,36.83 107.09,35.81 ARDUINO_DUE1.25
D26
  Bottom 0.305: ARDUINO_DUE1.26 96.41,39.64 98.74,39.64
  Bottom 0.406: 98.74,39.64 107.11,39.64 108.11,40.64 SV6.8
D27
  Bottom 0.406: ARDUINO_DUE1.27 107.09,38.35 108.11,39.37 110.49,39.37 SV6.7
D28
  Bottom 0.305: ARDUINO_DUE1.28 96.38,42.15 98.74,42.15
  Bottom 0.406: 98.74,42.15 107.08,42.15 108.11,43.18 SV6.10
D29
  Bottom 0.406: ARDUINO_DUE1.29 107.09,40.89 108.11,41.91 110.49,41.91 SV6.9
D30
  Bottom 0.305: ARDUINO_DUE1.30 96.41,44.72 98.74,44.72
  Bottom 0.406: 98.74,44.72 107.11,44.72 108.11,45.72 SV6.12
D31
  Bottom 0.406: ARDUINO_DUE1.31 107.09,43.43 108.11,44.45 110.49,44.45 SV6.11
D32
  Bottom 0.305: ARDUINO_DUE1.32 96.41,47.26 98.74,47.26
  Bottom 0.406: 98.74,47.26 107.11,47.26 108.11,48.26 SV6.14
D33
  Bottom 0.406: ARDUINO_DUE1.33 107.09,45.97 108.11,46.99 110.49,46.99 SV6.13
D34
  Bottom 0.305: ARDUINO_DUE1.34 96.41,49.8 98.74,49.8
  Bottom 0.406: 98.74,49.8 107.11,49.8 108.11,50.8 SV6.16
D35
  Bottom 0.406: ARDUINO_DUE1.35 107.09,48.51 108.11,49.53 110.49,49.53 SV6.15
D36
  Bottom 0.305: ARDUINO_DUE1.36 96.41,52.34 98.74,52.34
  Bottom 0.406: 98.74,52.34 107.11,52.34 108.11,53.34 SV6.18
D37
  Bottom 0.406: ARDUINO_DUE1.37 107.09,51.05 108.11,52.07 110.49,52.07 SV6.17
D38
  Bottom 0.305: ARDUINO_DUE1.38 96.38,54.85 98.74,54.85
  Bottom 0.406: 98.74,54.85 107.08,54.85 108.11,55.88 SV6.20
D39
  Bottom 0.406: ARDUINO_DUE1.39 107.09,53.59 108.11,54.61 110.49,54.61 SV6.19
D40
  Bottom 0.305: ARDUINO_DUE1.40 96.38,57.39 98.74,57.39
  Bottom 0.406: 98.74,57.39 107.08,57.39 108.11,58.42 SV6.22
D41
  Bottom 0.406: ARDUINO_DUE1.41 107.09,56.13 108.11,57.15 110.49,57.15 SV6.21
D42
  Bottom 0.305: ARDUINO_DUE1.42 96.38,59.93 98.74,59.93
  Bottom 0.406: 98.74,59.93 107.08,59.93 108.11,60.96 SV6.24
D43
  Bottom 0.406: ARDUINO_DUE1.43 107.09,58.67 108.11,59.69 110.49,59.69 SV6.23
D44
  Bottom 0.305: ARDUINO_DUE1.44 96.41,62.5 98.74,62.5
  Bottom 0.406: 98.74,62.5 107.11,62.5 108.11,63.5 SV6.26
D45
  Bottom 0.406: ARDUINO_DUE1.45 107.09,61.21 108.11,62.23 110.49,62.23 SV6.25
D46
  Bottom 0.305: ARDUINO_DUE1.46 96.41,65.04 98.74,65.04
  Bottom 0.406: 98.74,65.04 107.11,65.04 108.11,66.04 SV6.28
D47
  Bottom 0.406: ARDUINO_DUE1.47 107.09,63.75 108.11,64.77 110.49,64.77 SV6.27
D48
  Bottom 0.305: ARDUINO_DUE1.48 96.41,67.58 98.74,67.58
  Bottom 0.406: 98.74,67.58 107.11,67.58 108.11,68.58 SV6.30
D49
  Bottom 0.406: ARDUINO_DUE1.49 107.09,66.29 108.11,67.31 110.49,67.31 SV6.29
D50
  Bottom 0.305: ARDUINO_DUE1.50 96.38,70.09 98.74,70.09
  Bottom 0.406: 98.74,70.09 107.08,70.09 108.11,71.12 SV6.32
D51
  Bottom 0.406: ARDUINO_DUE1.51 107.09,68.83 108.11,69.85 110.49,69.85 SV6.31
D52
  Bottom 0.305: ARDUINO_DUE1.52 96.41,72.66 98.74,72.66
  Bottom 0.406: 98.74,72.66 107.11,72.66 108.11,73.66 SV6.34
D53
  Bottom 0.406: ARDUINO_DUE1.53 107.09,71.37 108.11,72.39 110.49,72.39 SV6.33
GND  (via drill 1 pad 1.93)
  Top 0.61: v26.67,25.72 22.23,25.72 21.43,24.92 21.43,20 | v41.91,82.71 26.83,82.71 26.04,83.5 26.04,90.65 25.24,91.44 15.88,91.44 | D2.A 15.88,91.44 | 15.88,91.44 1.75,91.44 1.11,90.81 1.11,20.8 1.91,20 21.43,20 | v52.07,106.52 45.72,106.52 44.93,105.73 44.93,96.36 44.07,95.5 v40.8,95.5 | 21.43,20 21.43,11.59 v20.32,10.48
  Bottom 0.406: ARDUINO_DUE1.GND_4 27.56,29.53 26.67,28.64 v26.67,25.72 SV2.2
  Bottom 0.61: 35.56,1.59 20.95,1.59 20.32,2.22 J18.1 v20.32,10.48 | 35.56,1.59 J15.1 35.56,14.92 36.2,15.56 41.27,15.56 41.91,16.19 SV16.8 | SV16.1 SV16.2 SV16.3 SV16.4 SV16.5 SV16.6 SV16.7 SV16.8 | SV16.8 SV10.1 SV10.2 SV10.3 SV10.4 SV10.5 SV10.6 SV10.7 SV10.8 SV11.1 SV11.2 SV11.3 SV11.4 SV11.5 SV11.6 SV11.7 SV11.8 | C5.2 J4.3 55.88,1.59 | C4.2 J3.3 66.04,1.59 | 35.56,1.59 50.8,1.59 | 50.8,1.59 55.88,1.59 | 55.88,1.59 66.04,1.59 | 66.04,1.59 76.2,1.59 | 76.2,1.59 86.36,1.59 | J5.4 86.36,1.59 | 76.2,1.59 J2.3 C3.2 | J16.1 50.8,1.59 | J1.2 101.6,1.59 | 101.6,1.59 86.36,1.59 | 101.6,1.59 108.9,1.59 109.54,2.22 109.54,9.53 110.17,10.16 113.67,10.16 114.3,10.79 SV1.10 119.06,15.24 119.7,15.88 119.7,32.38 119.06,33.02 SV9.1 SV9.3 SV9.5 SV9.7 SV9.9 SV9.11 SV9.13 SV9.15 SV9.17 SV9.19 SV9.21 SV9.23 SV9.25 SV9.27 SV9.29 SV9.31 SV9.33 SV9.35 119.06,76.2 119.7,76.83 119.7,96.52 118.9,97.31 113.67,97.31 113.03,96.68 J13.2 J14.2 | X1.2 5.08,91.44 4.37,90.73 S1.4 S1.3 13.37,88.62 13.65,88.9 C8.2 | C8.2 15.24,91.76 15.88,92.39 D2.A 15.88,96.2 16.32,96.65 C2.- 22.35,95.89 C1.2 31.43,95.89 31.81,95.5 U1.IN- v40.8,95.5 44.07,95.5 44.93,96.36 44.93,109.06 45.56,109.7 77.63,109.7 79.69,111.76 J6.3 | J8.2 16.51,87.63 C8.2 | J11.2 J12.2 104.14,76.2 | J9.2 J10.2 93.98,91.44 SV17.8 SV17.7 SV17.6 SV17.5 SV17.4 SV17.3 SV17.2 SV17.1 | SV7.6 v41.91,82.71 41.91,79.12 ARDUINO_DUE1.GND | SV7.7 44.45,79.12 ARDUINO_DUE1.GND_1 ARDUINO_DUE1.GND | U1.OUT- 74.93,93.47 SV17.1 | J7.3 C7.2 80.26,95.5 U1.OUT- | SV17.1 SV15.8 SV15.7 SV15.6 SV15.5 SV15.4 SV15.3 SV15.2 SV15.1 | SV6.35 SV6.36 104.14,76.2 | 104.14,76.2 101.85,73.91 ARDUINO_DUE1.GND_3 ARDUINO_DUE1.GND_2 91.69,73.91 91.12,73.34 91.12,70.8 90.49,70.17 42.55,70.17 41.75,70.96 41.75,78.96 ARDUINO_DUE1.GND
  Bottom 0.61: 76.96,106.65 76.99,106.68 C6.2 | U1.OUT- 76.96,106.65 | 76.96,106.65 52.2,106.65 v52.07,106.52
  pour Top (isolate 0.406, hatched): 122,3.41 122,115 arc90 119,118 3.41,118 arc90 0,114.59 0,3.41 arc90 3.41,0 118.59,0 arc90
  pour Bottom (isolate 0.406, hatched): 122,3.41 122,115 arc90 119,118 3.41,118 arc90 0,114.59 0,3.41 arc90 3.41,0 118.59,0 arc90
L1_DIR
  Bottom 0.406: SV2.4 31.75,28.64 32.64,29.53 ARDUINO_DUE1.12 32.64,33.72 32.07,34.29 5.4,34.29 5.08,33.97 5.08,23.18 5.4,22.86 8.57,22.86 8.89,23.18 R7.1
L1_EN
  Bottom 0.406: R6.1 11.43,22.23 11.11,21.91 4.76,21.91 4.13,22.54 4.13,34.92 4.45,35.24 34.61,35.24 35.18,34.67 ARDUINO_DUE1.11 35.18,29.53 34.29,28.64 SV2.5
L1_MAX  (via drill 1 pad 1.93)
  Top 0.406: v64.77,81.44 64.77,83.19 65.32,83.74 96.04,83.74 96.52,84.21 v96.52,97.63
  Bottom 0.406: ARDUINO_DUE1.A5 64.64,80.17 64.77,80.3 v64.77,81.44 SV5.6 | J10.1 v96.52,97.63
L1_MIN  (via drill 1 pad 1.93)
  Top 0.406: v62.23,81.44 62.23,83.19 61.75,83.66 50.64,83.66 50.01,84.3 50.01,97 50.64,97.63 v52.07,97.63 | v52.07,101.76 53.98,101.76 54.77,100.97 76.68,100.97 77.31,101.6 77.31,107.63 77.79,108.11 86.84,108.11 87.15,107.79 v96.52,107.79
  Bottom 0.406: ARDUINO_DUE1.A4 62.1,80.17 62.23,80.3 v62.23,81.44 SV5.5 | J9.1 v96.52,107.79 | v52.07,97.63 v52.07,101.76
L1_STEP
  Bottom 0.406: R8.1 6.35,33.02 6.67,33.34 29.53,33.34 30.1,32.77 ARDUINO_DUE1.13 30.1,29.53 29.21,28.64 SV2.3
L2_DIR  (via drill 1 pad 1.93)
  Top 0.406: R10.1 16.51,22.23 16.19,21.91 4.76,21.91 4.13,22.54 4.13,33.97 4.45,34.29 35.88,34.29 36.83,35.24 39.69,35.24 40.32,34.61 v40.32,33.34
  Bottom 0.406: SV2.7 39.37,28.64 40.26,29.53 ARDUINO_DUE1.9 40.32,30.8 v40.32,33.34
L2_EN  (via drill 1 pad 1.93)
  Top 0.406: R9.1 19.05,21.27 18.73,20.95 4.13,20.95 3.17,21.91 3.17,34.92 3.49,35.24 35.24,35.24 36.2,36.2 42.23,36.2 42.86,35.56 v42.86,33.34
  Bottom 0.406: SV2.8 41.91,28.64 42.8,29.53 ARDUINO_DUE1.8 42.86,30.8 v42.86,33.34
L2_MAX  (via drill 1 pad 1.93)
  Top 0.406: v69.85,81.44 99.38,81.44 100.01,82.07 100.01,96.68 100.97,97.63 v106.68,97.63
  Bottom 0.406: ARDUINO_DUE1.A7 69.72,80.17 69.85,80.3 v69.85,81.44 SV5.8 | J12.1 v106.68,97.63
L2_MIN  (via drill 1 pad 1.93)
  Top 0.406: v106.68,107.79 99.54,107.79 99.06,107.31 99.06,83.5 98.58,83.03 67.63,83.03 67.31,82.71 v67.31,81.44
  Bottom 0.406: ARDUINO_DUE1.A6 67.18,80.17 67.31,80.3 v67.31,81.44 SV5.7 | J11.1 v106.68,107.79
L2_STEP  (via drill 1 pad 1.93)
  Top 0.406: R11.1 13.97,23.18 13.65,22.86 5.4,22.86 5.08,23.18 5.08,33.02 5.4,33.34 v37.78,33.34
  Bottom 0.406: SV2.6 36.83,28.64 37.72,29.53 ARDUINO_DUE1.10 37.78,30.8 v37.78,33.34
MEGA_PENDANT_RX  (via drill 1 pad 1.93)
  Top 0.406: v74.93,25.08 74.93,28.73 75.41,29.21 88.74,29.21 89.38,28.57 98.74,28.57 99.69,27.62 99.69,23.5 R15.1
  Bottom 0.406: ARDUINO_DUE1.16 74.8,29.53 74.93,29.4 v74.93,25.08 SV4.3
MEGA_PENDANT_TX  (via drill 1 pad 1.93)
  Top 0.406: R16.1 99.06,20.32 98.74,20.64 98.74,26.83 97.79,27.78 89.06,27.78 88.42,28.42 77.95,28.42 77.47,27.94 v77.47,25.08
  Bottom 0.406: ARDUINO_DUE1.17 77.34,29.53 77.47,29.4 v77.47,25.08 SV4.4
N$1
  Bottom 0.406: ARDUINO_DUE1.RESET 34.29,78.87 D1.A
N$2
  Bottom 1.27: X1.1 8.87,100.31 10.97,102.41 F1.1
N$3  (via drill 1 pad 1.93)
  Top 0.406: v83.82,11.43 83.82,15.56 83.5,15.88 68.58,15.88 68.26,16.19 68.26,40.32 67.94,40.64 60.01,40.64 59.69,40.96 R1.2
  Bottom 0.406: J2.1 83.19,6.35 83.82,6.99 v83.82,11.43
N$4  (via drill 1 pad 1.93)
  Top 0.406: v73.66,11.43 73.66,14.61 73.34,14.92 67.63,14.92 67.31,15.24 67.31,39.37 66.99,39.69 57.47,39.69 57.15,40.01 R2.2
  Bottom 0.406: v73.66,11.43 73.66,6.99 73.03,6.35 J3.1
N$5  (via drill 1 pad 1.93)
  Top 0.406: v63.5,11.43 63.5,15.24 63.82,15.56 66.04,15.56 66.36,15.88 66.36,38.42 66.04,38.73 54.93,38.73 54.61,39.05 R3.2
  Bottom 0.406: J4.1 62.87,6.35 63.5,6.99 v63.5,11.43
N$6
  Bottom 0.406: J5.2 91.44,11.75 91.76,12.06 93.66,12.06 93.98,12.38 R4.2
N$7
  Bottom 0.406: J5.3 88.9,12.38 89.22,12.7 91.12,12.7 91.44,13.02 R5.2
N$8
  Bottom 0.406: R6.2 11.43,13.65 11.75,13.34 17.46,13.34 17.78,13.02 J18.2
N$9
  Bottom 0.406: J18.3 15.24,12.06 14.92,12.38 9.21,12.38 8.89,12.7 R7.2
N$10
  Bottom 0.406: R8.2 6.35,11.75 6.67,11.43 12.38,11.43 12.7,11.11 J18.4
N$11
  Bottom 0.406: J15.2 33.02,15.88 32.7,16.19 20.95,16.19 20.64,16.51 R9.2
N$12
  Bottom 0.406: R10.2 16.51,15.56 16.83,15.24 30.16,15.24 30.48,14.92 J15.3
N$13
  Bottom 0.406: R11.2 13.97,14.61 14.29,14.29 27.62,14.29 27.94,13.97 J15.4
N$14  (via drill 1 pad 1.93)
  Top 0.406: v43.18,10.48 43.18,12.06 43.5,12.38 43.5,28.57 44.45,29.53 44.45,40.32 44.77,40.64 46.67,40.64 46.99,40.96 R14.2
  Bottom 0.406: J16.4 v43.18,10.48
N$15  (via drill 1 pad 1.93)
  Top 0.406: v45.72,10.48 45.72,12.06 44.45,13.34 44.45,28.26 45.4,29.21 45.4,39.37 45.72,39.69 49.21,39.69 49.53,40.01 R13.2
  Bottom 0.406: J16.3 v45.72,10.48
N$16  (via drill 1 pad 1.93)
  Top 0.305: 48.15,29.41 48.15,31.95
  Top 0.406: v48.26,10.48 48.26,12.06 45.4,14.92 45.4,27.94 46.04,28.57 47.31,28.57 48.15,29.41 | 48.15,31.95 48.26,32.07 48.26,38.42 48.58,38.73 51.75,38.73 52.07,39.05 R12.2
  Bottom 0.406: J16.2 v48.26,10.48
N$17
  Bottom 0.406: SV1.3 R15.2
N$18
  Bottom 0.406: SV1.5 R16.2
N$19
  Bottom 0.406: SV1.7 R17.2
N$20
  Bottom 0.406: SV1.9 R18.2
N$21  (via drill 3.2 pad 6)
  other vias: 5,113
N$22  (via drill 3.2 pad 6)
  other vias: 5,5
N$23  (via drill 3.2 pad 6)
  other vias: 117,5
N$24  (via drill 3.2 pad 6)
  other vias: 117,113
NEXTION_RX  (via drill 1 pad 1.93)
  Top 0.406: R17.1 98.11,17.78 97.79,18.1 97.79,26.04 96.84,26.99 88.74,26.99 88.11,27.62 80.49,27.62 80.01,27.15 v80.01,25.08
  Bottom 0.406: ARDUINO_DUE1.18 79.88,29.53 80.01,29.4 v80.01,25.08 SV4.5
NEXTION_TX  (via drill 1 pad 1.93)
  Top 0.406: R18.1 97.16,15.24 96.84,15.56 96.84,25.24 95.89,26.19 88.42,26.19 87.79,26.83 83.03,26.83 82.55,26.35 v82.55,25.08
  Bottom 0.406: ARDUINO_DUE1.19 82.42,29.53 82.55,29.4 v82.55,25.08 SV4.6
SCL
  Bottom 0.406: ARDUINO_DUE1.21 87.5,27.94 87.63,27.81 SV4.8 92.71,22.86 R4.1
SDA  (via drill 1 pad 1.93)
  Top 0.406: v85.09,25.08 90.49,25.08 R5.1
  Bottom 0.406: ARDUINO_DUE1.20 84.96,29.53 85.09,29.4 v85.09,25.08 SV4.7
SERVO1
  Bottom 0.406: SV3.6 59.69,27.81 59.56,27.94 ARDUINO_DUE1.2 59.56,31.75 59.69,31.88 R1.1
SERVO2
  Bottom 0.406: SV3.5 57.15,27.81 57.02,27.94 ARDUINO_DUE1.3 57.02,31.75 57.15,31.88 R2.1
SERVO3
  Bottom 0.406: SV3.4 54.61,27.81 54.48,27.94 ARDUINO_DUE1.4 54.48,31.75 54.61,31.88 R3.1
SW_EMRGNCY  (via drill 1 pad 1.93)
  Top 0.406: v118.11,25.4 118.11,13.97 117.79,13.65 99.38,13.65 99.06,13.34 J1.3
  Bottom 0.406: SV1.2 v118.11,25.4
TRIM_L1  (via drill 1 pad 1.93)
  Top 0.406: v79.06,104.93 79.06,100.97 78.26,100.17 49.21,100.17 48.42,99.38 48.42,82.07 49.05,81.44 v52.07,81.44
  Bottom 0.406: ARDUINO_DUE1.A0 51.94,80.2 52.07,80.33 v52.07,81.44 SV5.1 | J6.1 C6.1 84.61,104.93 v79.06,104.93
TRIM_L2  (via drill 1 pad 1.93)
  Top 0.406: v54.61,81.44 54.61,82.55 54.25,82.91 50.48,82.91 50.44,82.87 49.85,82.87 49.21,83.5 49.21,98.9 49.69,99.38 78.26,99.38 79.06,98.58 79.06,94.93 79.85,94.14 v81.28,94.14
  Bottom 0.406: J7.1 C7.1 86.36,95.25 85.25,94.14 v81.28,94.14 | ARDUINO_DUE1.A1 54.48,80.2 54.61,80.33 v54.61,81.44 SV5.2
VIN
  Bottom 0.61: ARDUINO_DUE1.VIN 46.99,79.12 SV7.8
Z_DIR
  Bottom 0.406: SV3.2 49.53,27.81 49.4,27.94 ARDUINO_DUE1.6 49.4,31.75 49.53,31.88 R13.1
Z_EN
  Bottom 0.406: SV3.3 52.07,27.81 51.94,27.94 ARDUINO_DUE1.5 51.94,31.75 52.07,31.88 R12.1
Z_MAX  (via drill 1 pad 1.93)
  Top 0.406: v77.47,75.04 79.49,75.04 79.85,75.41 107.31,75.41 107.79,75.88 107.79,79.22 108.27,79.69 v115.57,79.69
  Bottom 0.406: SV8.2 77.47,80.3 77.34,80.17 ARDUINO_DUE1.A9 77.34,75.17 v77.47,75.04 | J14.1 v115.57,79.69
Z_MIN  (via drill 1 pad 1.93)
  Top 0.406: v74.93,76.52 79.38,76.52 79.69,76.2 106.52,76.2 107,76.68 107,89.53 107.47,90.01 v115.57,90.01
  Bottom 0.406: SV8.1 74.93,80.3 74.8,80.17 ARDUINO_DUE1.A8 74.8,76.64 v74.93,76.52 | J13.1 v115.57,90.01
Z_STEP
  Bottom 0.406: SV3.1 46.99,27.81 46.86,27.94 ARDUINO_DUE1.7 46.86,31.75 46.99,31.88 R14.1

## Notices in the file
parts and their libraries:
diy-modules: Released under the Creative Commons Attribution 4.0 International License: http://creativecommons.org/licenses/by/4.0
